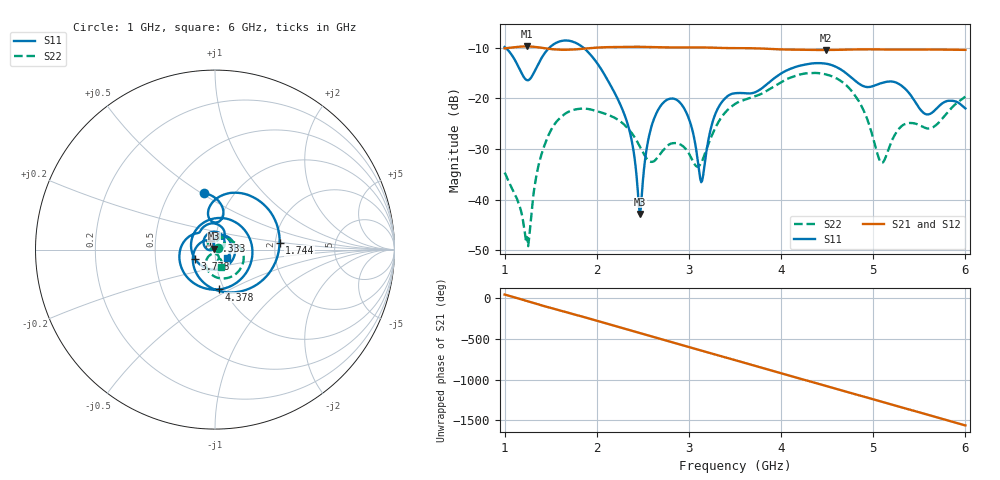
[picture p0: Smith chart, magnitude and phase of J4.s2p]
!Agilent Technologies,E8364B,MY43040528,A.07.50.67
!Agilent E8364B: A.07.50.67
!Date: Sunday, March 01, 2026 15:24:33
!Correction: S11(Full 2 Port(1,2))
!S21(Full 2 Port(1,2))
!S12(Full 2 Port(1,2))
!S22(Full 2 Port(1,2))
!S2P File: Measurements: S11, S21, S12, S22:
# Hz S  dB  R 50
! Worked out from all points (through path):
!   451 points, 1 GHz to 6 GHz, reference 50 ohm
!   highest |S21| = -9.74 dB at 1.244 GHz (marker M1); lowest = -10.4 dB at 4.489 GHz (marker M2)
!   group delay of S21, straight-line fit = 892 ps
!   lowest |S11| = -42.8 dB at 2.467 GHz (marker M3), VSWR 1.01, Z = 49.5 + j0.517 ohm
!   |S11| at or under -10 dB: 1.01 GHz to 1.485 GHz (475.6 MHz wide, 38.1 % of centre); 1.856 GHz to end of sweep
!   |S22| runs from -49.1 to -15.0 dB; largest |S21 - S12| = 0.0014
!   S11 on the Smith chart (normalised r, x): 1 GHz: 0.73, +0.51; 1.744 GHz: 2.11, +0.18; 2.333 GHz: 0.95, +0.10; 3.778 GHz: 0.79, -0.08; 4.378 GHz: 0.94, -0.44; 6 GHz: 1.14, -0.10
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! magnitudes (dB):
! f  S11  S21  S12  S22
! 1 GHz  -9.9  -10.1  -10.1  -34.6
! 1.244 GHz  -16.4  -9.7  -9.8  -47.4
! 1.433 GHz  -11.1  -10.1  -10.1  -29.2
! 1.744 GHz  -8.8  -10.3  -10.4  -22.3
! 1.844 GHz  -9.8  -10.2  -10.2  -22.0
! 2.333 GHz  -24.9  -9.8  -9.8  -25.8
! 2.467 GHz  -42.8  -9.8  -9.8  -29.5
! 2.556 GHz  -28.5  -9.8  -9.9  -32.2
! 2.667 GHz  -22.2  -9.9  -9.9  -31.5
! 2.933 GHz  -21.5  -9.9  -10.0  -29.4
! 3.133 GHz  -36.5  -9.9  -10.0  -32.7
! 3.289 GHz  -23.0  -10.0  -10.0  -25.7
! 3.5 GHz  -19.0  -10.1  -10.1  -21.1
! 3.778 GHz  -18.2  -10.1  -10.2  -19.2
! 4.344 GHz  -13.1  -10.4  -10.5  -15.0
! 4.378 GHz  -13.0  -10.4  -10.5  -15.0
! 4.489 GHz  -13.1  -10.4  -10.5  -15.3
! 4.833 GHz  -16.9  -10.3  -10.4  -20.2
! 5.078 GHz  -17.0  -10.3  -10.4  -32.5
! 5.167 GHz  -16.7  -10.4  -10.4  -30.0
! 5.567 GHz  -23.1  -10.3  -10.4  -25.8
! 6 GHz  -22.0  -10.4  -10.4  -19.6
